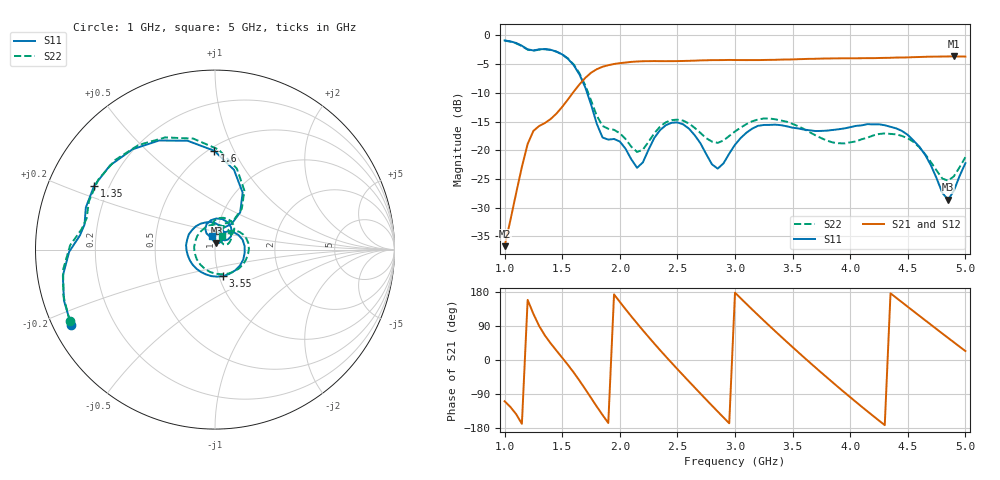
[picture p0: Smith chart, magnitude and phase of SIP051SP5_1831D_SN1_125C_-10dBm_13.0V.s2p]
# GHz  S  dB  R  50
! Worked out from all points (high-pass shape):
!   81 points, 1 GHz to 5 GHz, reference 50 ohm
!   highest |S21| = -3.65 dB at 4.9 GHz (marker M1); lowest = -36.7 dB at 1 GHz (marker M2)
!   |S21| within 3 dB of the highest: 1.742 GHz to end of sweep
!   lowest |S11| = -28.6 dB at 4.85 GHz (marker M3), VSWR 1.08, Z = 50.7 + j3.67 ohm
!   |S11| at or under -10 dB: 1.716 GHz to end of sweep
!   |S22| runs from -25.3 to -0.9 dB; largest |S21 - S12| = 0.0027
!   S11 on the Smith chart (normalised r, x): 1 GHz: 0.05, -0.24; 1.35 GHz: 0.14, +0.24; 1.6 GHz: 0.53, +0.84; 3.55 GHz: 1.05, -0.32; 5 GHz: 0.95, +0.14
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1  -0.87 -152.4  -36.71 -108.8  -36.63 -109.6  -0.89 -153.9
1.2  -2.42 174.0  -18.91 158.7  -18.88 158.7  -2.48 171.3
1.35  -2.37 152.2  -15.26 64.7  -15.23 64.6  -2.40 149.1
1.6  -5.18 90.4  -9.79 -33.0  -9.80 -33.1  -5.07 87.9
1.7  -9.04 64.2  -7.40 -76.8  -7.39 -76.7  -8.69 63.6
1.8  -15.39 57.2  -5.88 -122.8  -5.87 -122.7  -13.98 57.5
1.95  -18.04 81.1  -4.97 173.2  -5.00 173.2  -16.45 72.4
2.15  -23.05 94.4  -4.54 96.6  -4.53 96.7  -20.30 80.6
2.35  -16.47 108.0  -4.48 25.9  -4.47 26.0  -15.86 91.5
2.5  -15.15 76.3  -4.47 -24.1  -4.46 -24.1  -14.67 67.4
2.7  -18.78 39.5  -4.35 -88.6  -4.35 -88.6  -16.99 43.1
2.85  -23.20 53.7  -4.30 -136.0  -4.30 -136.1  -18.71 47.4
3  -19.04 60.3  -4.28 177.7  -4.27 177.7  -16.73 46.8
3.3  -15.58 -5.9  -4.26 89.8  -4.26 89.8  -14.46 2.0
3.55  -16.20 -72.6  -4.14 20.2  -4.13 20.2  -15.83 -49.5
3.7  -16.66 -110.5  -4.07 -20.2  -4.06 -20.2  -17.42 -88.2
4  -15.98 -178.4  -3.97 -98.1  -3.98 -98.1  -18.62 173.9
4.35  -15.92 108.7  -3.89 176.0  -3.90 176.0  -17.16 78.5
4.6  -19.38 61.8  -3.76 116.8  -3.75 116.8  -19.48 32.9
4.85  -28.63 77.8  -3.66 58.2  -3.67 58.3  -25.30 43.3
4.9  -27.05 96.3  -3.65 46.7  -3.66 46.6  -24.54 55.5
5  -22.25 103.7  -3.68 23.7  -3.68 23.6  -21.21 63.1
